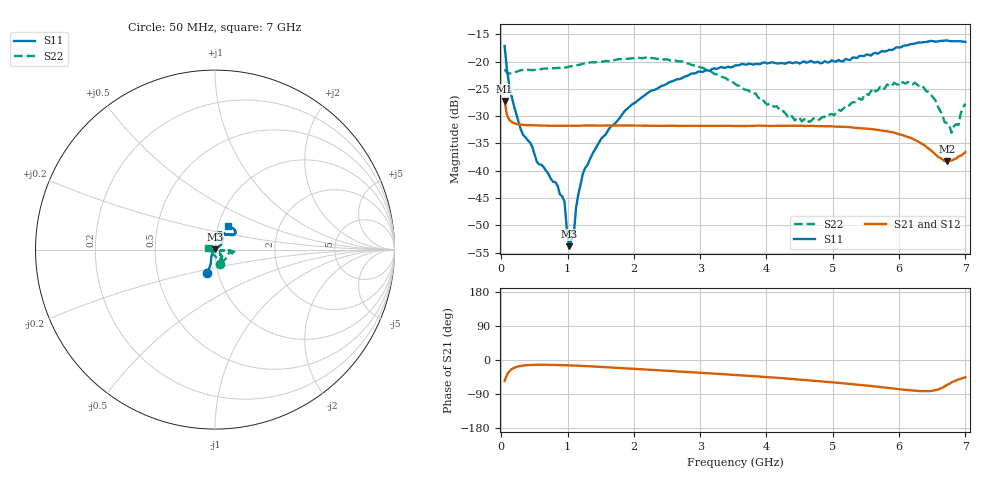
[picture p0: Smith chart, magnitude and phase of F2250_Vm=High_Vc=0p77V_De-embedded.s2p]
! Integrated Device Technology
! Corporate Headquarters
! 6024 Silver Creek Valley Road
! San Jose, CA 95138  USA
! Phone:  1-408-284-8200
! Toll Free:  1-800-223-1366
! Webpage:  http://www.idt.com/
! Timing and RF Division
! 515 Groton Road, Suite 102
! Westford, MA 01886-6024
! Device:  F2250
! Description: Voltage Variable RF Attenuator
! Frequency:  50.0 -  6000.00 MHz
! Package:  3x3 mm Thin QFN Plastic Package: 16 pin
! Ports:  2 RF, 3 DC
!  Pin  1  = GND
!  Pin  2  = NC
!  Pin  3  = RF1  = Port 1
!  Pin  4  = NC
!  Pin  5  = GND
!  Pin  6  = GND
!  Pin  7  = GND
!  Pin  8  = GND
!  Pin  9  = NC
!  Pin 10  = RF2  = Port 2
!  Pin 11  = NC
!  Pin 12  = GND
!  Pin 13  = GND
!  Pin 14  = VCNTRL
!  Pin 15  = VDD
!  Pin 16  = VMODE
! Vcntrl:  0.770 Volts
! Vmode:  +3.300 Volts
! Vdd:  +3.30  Volts
! Current:  1.297 mA
! Data:  The device was measured on a the F2250 evaluation board which has
!  individual transmission lines to the RF pins.  Data was collected
!  using a calibrated network analyzer.  The evaluation board was
!  de-embedded using a TRL calibration technique.
!  The reference plane is the edge of the package pin.
! Misc:  SN 10
!  Action Tracker AT0258
! Date Measured:  2014-11-26
! Date:  2015-10-15  MJV
! Note:
!  Integrated Device Technology supplies this data as a sample of measured
!  data at the package pin for this product.  Your particular data for this
!  product may vary.
!  Data was taken at 25 degrees C.
!  Integrated Device Technology reserves the right to change this data at anytime.
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# GHz S dB R 50
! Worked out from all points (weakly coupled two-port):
!   201 points, 50 MHz to 7 GHz, reference 50 ohm
!   highest |S21| = -27.20 dB at 50 MHz (marker M1); lowest = -38.2 dB at 6.722 GHz (marker M2)
!   lowest |S11| = -53.8 dB at 1.023 GHz (marker M3), VSWR 1.00, Z = 49.9 + j0.153 ohm
!   |S11| at or under -10 dB: start of sweep to end of sweep
!   |S22| runs from -33.1 to -19.3 dB; largest |S21 - S12| = 9.6e-05
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0.05  -17.15 -107.8  -27.20 -55.5  -27.19 -55.4  -21.40 -69.8
0.1195  -24.20 -111.0  -30.65 -30.0  -30.65 -30.0  -22.17 -23.3
0.29325  -32.41 -125.4  -31.55 -15.6  -31.55 -15.6  -21.57 -11.5
0.467  -35.59 -143.6  -31.66 -12.9  -31.67 -12.9  -21.58 -7.8
0.5365  -38.36 -151.7  -31.69 -12.6  -31.70 -12.6  -21.44 -8.3
0.8145  -42.05 170.6  -31.75 -13.0  -31.74 -13.0  -21.22 -9.8
0.9535  -45.62 173.2  -31.75 -13.7  -31.75 -13.7  -21.11 -11.0
1.023  -53.81 131.3  -31.76 -14.1  -31.77 -14.1  -20.91 -10.9
1.0925  -51.95 68.6  -31.74 -14.6  -31.76 -14.6  -20.81 -11.1
1.12725  -46.76 49.7  -31.75 -14.8  -31.77 -14.8  -20.70 -11.5
1.2315  -40.46 35.7  -31.72 -15.6  -31.72 -15.6  -20.38 -12.7
1.6485  -31.92 39.2  -31.70 -19.6  -31.72 -19.6  -19.86 -11.8
2.37825  -24.75 45.8  -31.76 -27.1  -31.77 -27.1  -19.44 -8.8
3.525  -20.71 71.3  -31.79 -39.5  -31.78 -39.5  -24.06 -5.3
4.4285  -20.16 74.4  -31.73 -50.6  -31.75 -50.6  -30.78 -14.4
4.7065  -20.13 71.7  -31.78 -54.6  -31.79 -54.5  -30.40 -24.7
5.85325  -17.83 40.3  -32.85 -74.0  -32.85 -74.1  -24.49 -49.3
6.33975  -16.50 40.5  -35.00 -82.1  -35.01 -82.2  -24.43 -63.6
6.722  -16.13 49.1  -38.25 -65.7  -38.23 -65.8  -31.25 -115.8
6.7915  -16.28 51.1  -38.12 -59.0  -38.15 -58.9  -33.05 -136.8
6.89575  -16.25 56.2  -37.39 -51.3  -37.38 -51.3  -31.59 -171.1
7  -16.38 62.1  -36.56 -45.8  -36.52 -46.1  -27.72 169.0
